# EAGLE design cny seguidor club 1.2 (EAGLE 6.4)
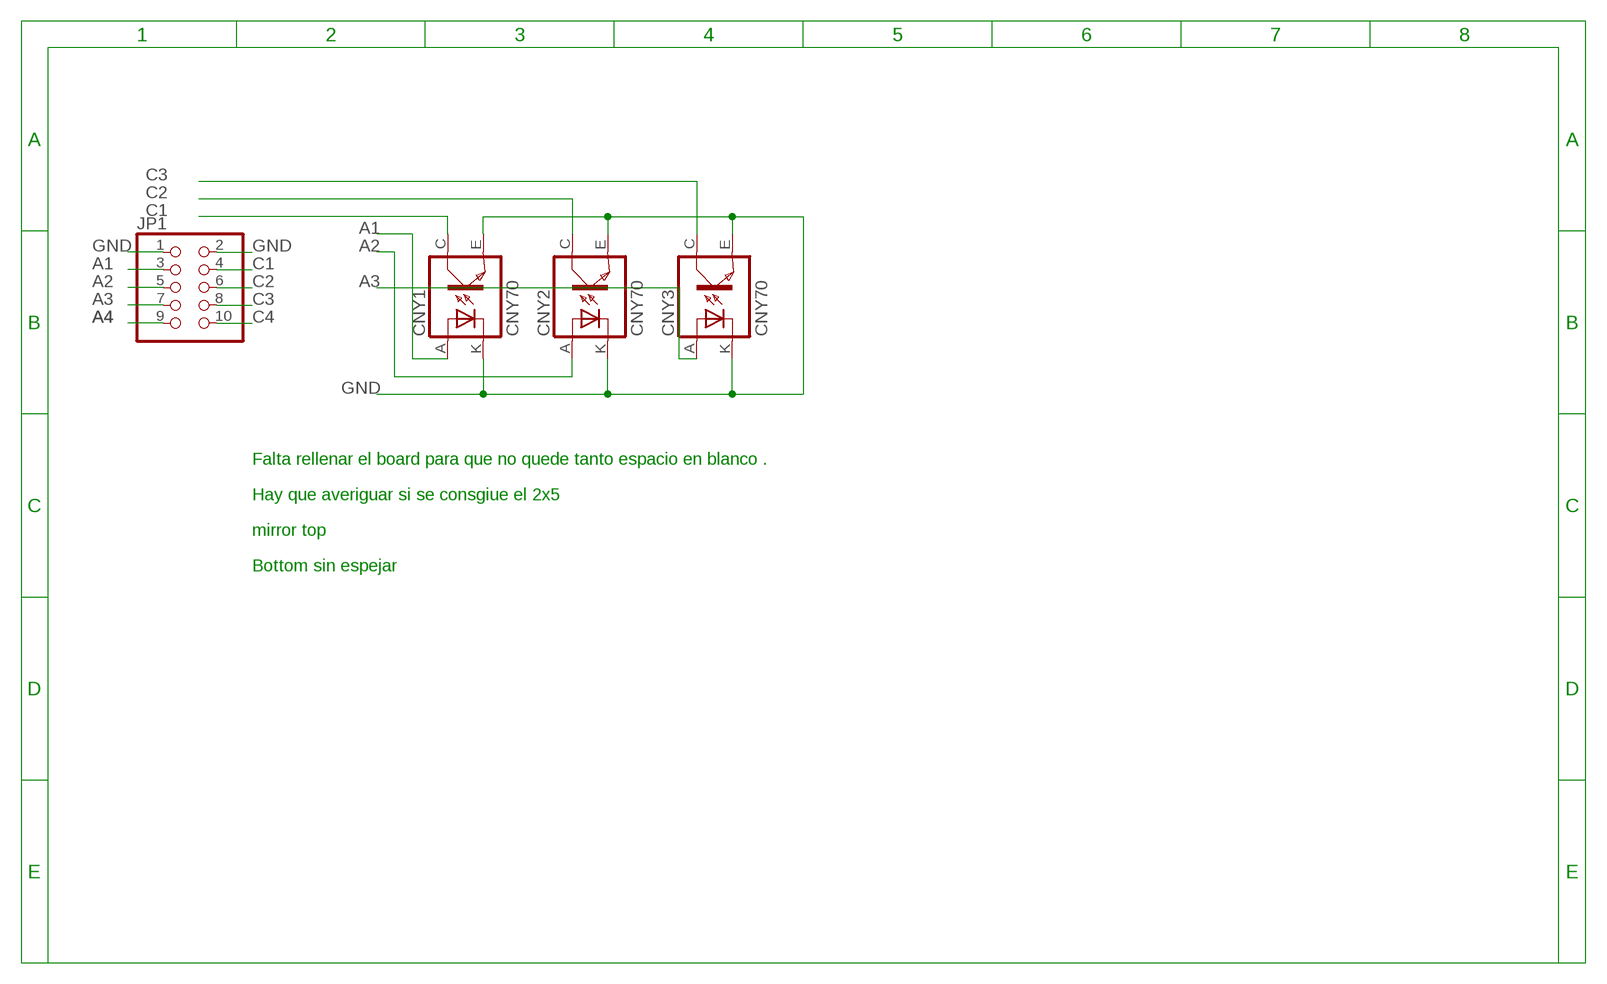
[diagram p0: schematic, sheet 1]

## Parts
CNY1  CNY70  [4]
CNY2  CNY70  [4]
CNY3  CNY70  [4]
JP1  PINHD-2X5/90  [2X05/90]

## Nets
A1: CNY1.A JP1.3
A2: CNY2.A JP1.5
A3: CNY3.A JP1.7
A4: JP1.9
C1: CNY1.C(COL) JP1.4
C2: CNY2.C(COL) JP1.6
C3: CNY3.C(COL) JP1.8
C4: JP1.10
GND: CNY1.E(EMI) CNY1.K(C) CNY2.E(EMI) CNY2.K(C) CNY3.E(EMI) CNY3.K(C) JP1.1 JP1.2

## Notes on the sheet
- Falta rellenar el board para que no quede tanto espacio en blanco .
- Hay que averiguar si se consgiue el 2x5
- mirror top
- Bottom sin espejar

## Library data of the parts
CNY1-CNY3 = cny70:CNY70
JP1 = pinhead:PINHD-2X5: PIN HEADER

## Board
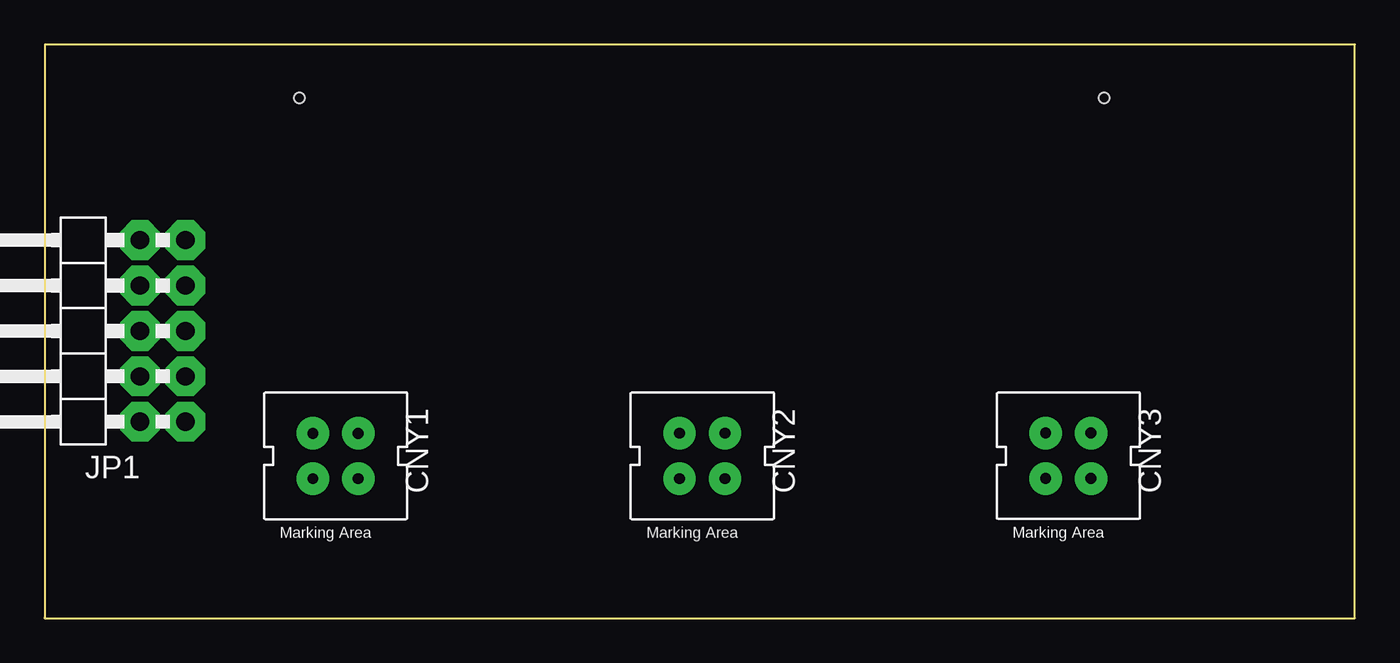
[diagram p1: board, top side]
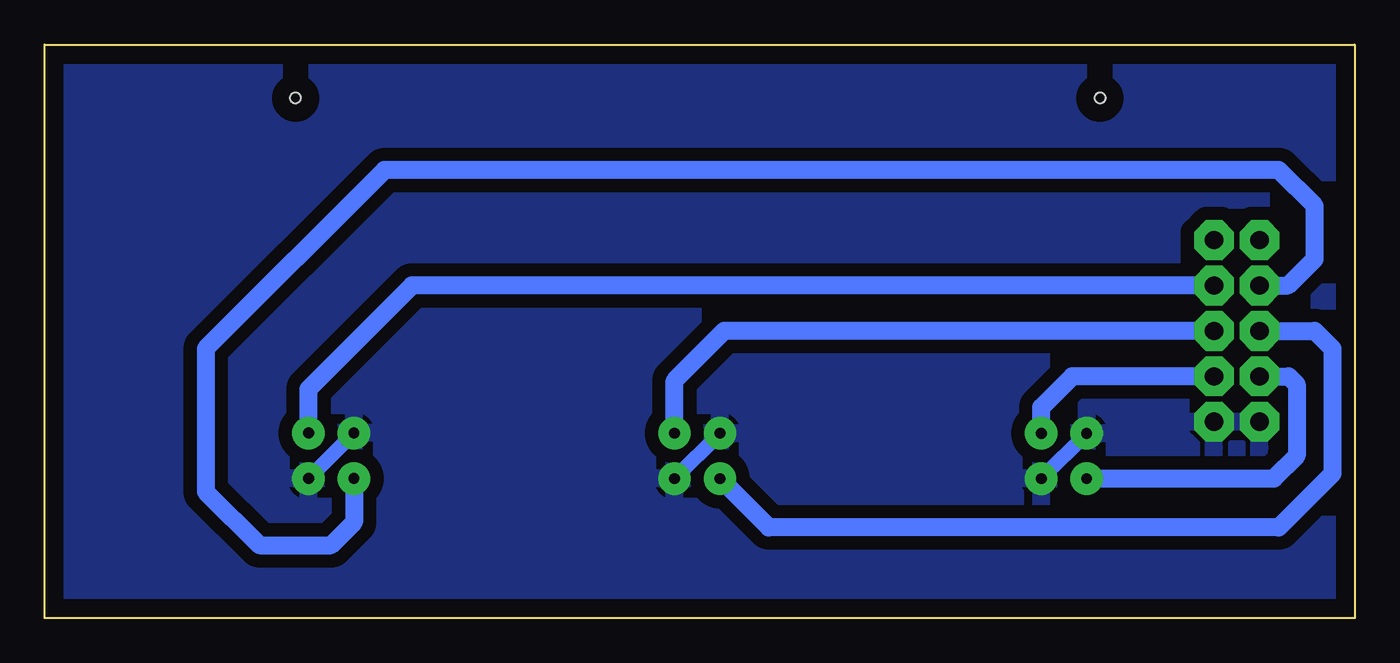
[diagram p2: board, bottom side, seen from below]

Size 73.26 x 32.09 mm. Coordinates in mm from the lower left corner, seen from the top.
Outline: 0,0 73.26,0 73.26,32.09 0,32.09 0,0
Copper layers (1*16): Top 0.035mm / dielectric 1.5mm / Bottom 0.035mm
Design rules "default *": minimum track width 0.5mm, minimum drill 0.01mm, track to track 0.75mm, track to pad 0.75mm, pad to pad 0.75mm, via to via 0.75mm, smd to smd 1mm, copper to edge 40mil, drill to drill 10mil, minimum pad ring 0.6mm, minimum via ring 0.75mm, stop-mask expansion 4mil, vias tented up to drill 0mil, thermal gap 10mil
Holes 0.6 mm at 59.23,29.1 14.25,29.1

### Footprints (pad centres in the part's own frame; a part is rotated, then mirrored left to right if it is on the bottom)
4 = drill 0.61 pad 1.27: A -1.27,1.27; C 1.27,-1.27; E 1.27,1.27; K -1.27,-1.27
2X05/90 = drill 1.016 octagon: 1 -5.08,-6.35; 2 -5.08,-3.81; 3 -2.54,-6.35; 4 -2.54,-3.81; 5 0,-6.35; 6 0,-3.81; 7 2.54,-6.35; 8 2.54,-3.81; 9 5.08,-6.35; 10 5.08,-3.81

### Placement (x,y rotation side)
CNY1  16.26,9.08 270 top
CNY2  36.77,9.08 270 top
CNY3  57.24,9.09 270 top
JP1  1.52,16.07 90 top

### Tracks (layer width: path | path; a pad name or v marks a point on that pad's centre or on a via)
A1
  Bottom 1: JP1.3 15.8,13.53 17.53,11.8 CNY1.A
A2
  Bottom 1: JP1.5 35.26,16.07 38.04,13.3 CNY2.A
A3
  Bottom 1: CNY3.A 58.51,12.83 52.72,18.61 JP1.7
C1
  Bottom 1: JP1.4 3.7,13.53 3.25,13.08 3.25,9.08 4.52,7.81 CNY1.C
C2
  Bottom 1: CNY2.C 32.77,5.08 4.25,5.08 1.25,8.08 1.25,15.08 2.24,16.07 JP1.6
C3
  Bottom 1: JP1.8 3.72,18.61 2.25,20.08 2.25,23.08 4.25,25.08 54.25,25.08 64.25,15.08 64.25,7.08 61.25,4.08 57.25,4.08 55.97,5.37 CNY3.C
GND
  Bottom 0.8: CNY1.E CNY1.K | CNY2.E CNY2.K | CNY3.E CNY3.K
  pour Bottom (isolate 0.6): 0.21,-0.35 73.72,-0.35 73.72,31.8 -0.62,31.8 -0.62,-0.24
